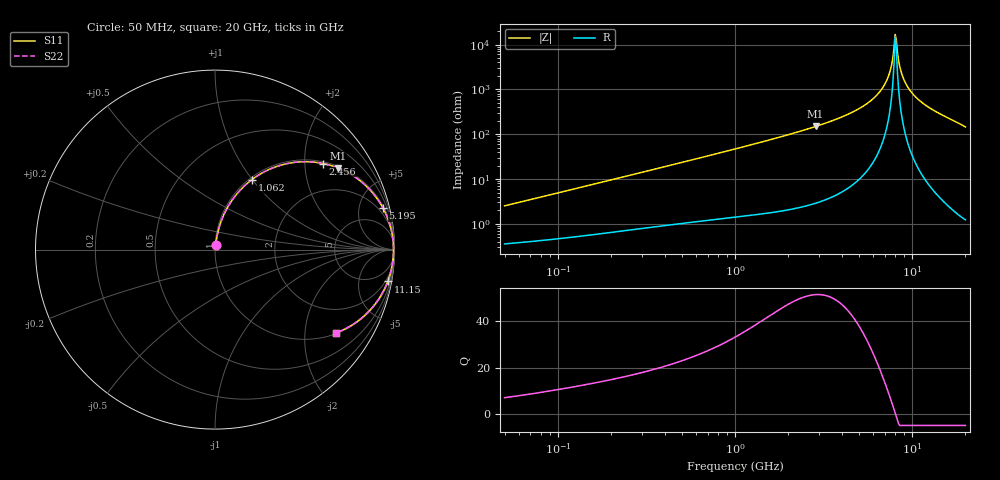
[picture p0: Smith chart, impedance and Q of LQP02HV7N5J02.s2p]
!Murata Part Number: LQP02HV7N5J02
!These Parameters are Measured in Series Mode Connection
!  o--[Z]--o
!Port1  Port2
!  o-------o
!Freq. Start=50[MHz] Stop=20[GHz], 401[Steps]
# Hz S RI R 50
!Freq.(Hz) S11(Real) S11(Imag) S21(Real) S21(Imag) S12(Real) S12(Imag) S22(Real) S22(Imag)
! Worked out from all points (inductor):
!   401 points, 50 MHz to 20 GHz, reference 50 ohm
!   read as one part in series: L = 7.88 nH near 51.52 MHz
!   highest Q = 51.5 at 2.853 GHz (marker M1), where L = 8.29 nH
!   self-resonance near 8.021 GHz
!   S11 on the Smith chart (normalised r, x): 50 MHz: 1.01, +0.05; 1.062 GHz: 1.03, +0.99; 2.456 GHz: 1.05, +2.47; 5.195 GHz: 1.22, +8.06; 11.15 GHz: 1, -11; 20 GHz: 1.02, -2.90
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5e7  0.00417 0.0248  0.9958 -0.0248  0.9958 -0.0248  0.00417 0.0248
1.364002e8  0.00957 0.0649  0.9904 -0.0649  0.9904 -0.0649  0.00957 0.0649
3.721004e8  0.0377 0.1669  0.9623 -0.1669  0.9623 -0.1669  0.0377 0.1669
1e9  0.1866 0.3748  0.8134 -0.3748  0.8134 -0.3748  0.1866 0.3748
1.061746e9  0.2049 0.3893  0.7951 -0.3893  0.7951 -0.3893  0.2049 0.3893
2.456456e9  0.6022 0.4796  0.3978 -0.4796  0.3978 -0.4796  0.6022 0.4796
2.728004e9  0.6607 0.4638  0.3393 -0.4638  0.3393 -0.4638  0.6607 0.4638
2.853386e9  0.6853 0.4548  0.3147 -0.4548  0.3147 -0.4548  0.6853 0.4548
5.194772e9  0.9363 0.2307  0.0637 -0.2307  0.0637 -0.2307  0.9363 0.2307
6.503449e9  0.9805 0.1157  0.0195 -0.1157  0.0195 -0.1157  0.9805 0.1157
7.009217e9  0.9886 0.0757  0.0114 -0.0757  0.0114 -0.0757  0.9886 0.0757
7.442007e9  0.9926 0.0434  0.00737 -0.0434  0.00737 -0.0434  0.9926 0.0434
7.668323e9  0.9939 0.0272  0.00614 -0.0272  0.00614 -0.0272  0.9939 0.0272
7.901521e9  0.9946 0.0109  0.00544 -0.0109  0.00544 -0.0109  0.9946 0.0109
8.141811e9  0.9947 -0.00548  0.00529 0.00548  0.00529 0.00548  0.9947 -0.00548
8.264682e9  0.9946 -0.0137  0.00541 0.0137  0.00541 0.0137  0.9946 -0.0137
8.644534e9  0.9934 -0.0382  0.00661 0.0382  0.00661 0.0382  0.9934 -0.0382
9.041845e9  0.991 -0.0629  0.00904 0.0629  0.00904 0.0629  0.991 -0.0629
9.892087e9  0.9823 -0.112  0.0177 0.112  0.0177 0.112  0.9823 -0.112
1.115139e10  0.9626 -0.1772  0.0374 0.1772  0.0374 0.1772  0.9626 -0.1772
1.396067e10  0.898 -0.2957  0.102 0.2957  0.102 0.2957  0.898 -0.2957
2e10  0.6761 -0.4637  0.3239 0.4637  0.3239 0.4637  0.6761 -0.4637
